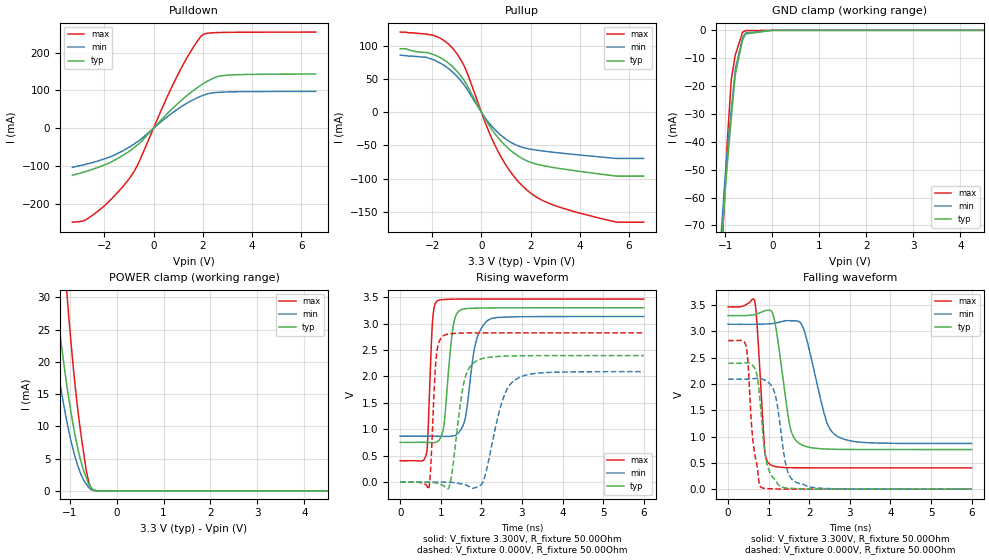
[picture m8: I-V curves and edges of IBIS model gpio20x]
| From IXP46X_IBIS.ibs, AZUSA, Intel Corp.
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[Model]   gpio20x
Model_type   I/O
Vinl = 800.000mV
Vinh = 2.000V
Vmeas = 1.500V
Cref = 0.000F
|   typ   min   max
C_comp   3.000pF   2.700pF   3.300pF
[Voltage Range]   3.300V   3.135V   3.465V
[Temperature Range]   25.0   110.0   -40.0
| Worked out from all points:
|   slope of the pulldown table from 0 to 0.495 V, typ, clamps not added: 14.5 ohm
|   slope of the pullup table from 0 to 0.495 V, typ, clamps not added: 16.7 ohm
|   POWER clamp passes 1 mA (typ) near -0.59 V on its own axis
|   falling waveform, V_fixture 3.300V, R_fixture 50.00Ohm: 20-80 % time 276ps typ, 421ps min, 141ps max; typ from 3.3 V to 0.753 V
|   rising waveform, V_fixture 3.300V, R_fixture 50.00Ohm: 20-80 % time 173ps typ, 247ps min, 92.3ps max; typ from 0.753 V to 3.3 V
|   rising waveform, V_fixture 0.000V, R_fixture 50.00Ohm: 20-80 % time 254ps typ, 400ps min, 105ps max; typ from 0 V to 2.4 V
|   falling waveform, V_fixture 0.000V, R_fixture 50.00Ohm: 20-80 % time 203ps typ, 243ps min, 179ps max; typ from 2.4 V to 0 V
[Pulldown]
|   Voltage   I(typ)   I(min)   I(max)
-3.3V     -124.6mA   -103.5mA   -248.9mA
-2.755V   -114.7mA   -95.53mA   -242.6mA
-2.29V    -104.7mA   -87.33mA   -221.2mA
-1.635V   -86.44mA   -72.55mA   -182.3mA
-925mV    -58.32mA   -47.76mA   -127.9mA
-605mV    -41.95mA   -33.66mA   -91.57mA
940mV     62.44mA    48.6mA     135.3mA
1.535V    95.49mA    72.67mA    205.6mA
1.99V     116.4mA    86.38mA    247mA
2.545V    135.5mA    94.53mA    253.1mA
2.875V    139.7mA    95.72mA    253.6mA
6.595V    143.5mA    97.58mA    254.5mA
[GND Clamp]
|   Voltage   I(typ)   I(min)   I(max)
-3.3V     -1.837A    -1.782A    -2.189A
-1.11V    -85mA      -78.05mA   -94.07mA
-1.015V   -60.26mA   -54.83mA   -58.33mA
-985mV    -53.42mA   -48.7mA    -48.27mA
-960mV    -48.28mA   -43.8mA    -39.96mA
-875mV    -31.55mA   -28.61mA   -17.72mA
-785mV    -15.46mA   -13.66mA   -8.602mA
-635mV    -3.516mA   -2.727mA   -731.7uA
-580mV    -1.636mA   -1.201mA   -155.8uA
-565mV    -1.289mA   -945.2uA   -102.2uA
0V        -56.84nA   -17.58nA   -565.5pA
6.595V    0A         0A         0A
[Pullup]
|   Voltage   I(typ)   I(min)   I(max)
-3.3V     95.67mA    85.92mA    120.8mA
-1.9V     86.2mA     78.19mA    115.1mA
-1.07V    64.88mA    56.95mA    91.89mA
-630mV    43.49mA    37.35mA    63.71mA
215mV     -13.96mA   -11.5mA    -21.37mA
695mV     -39.16mA   -31.53mA   -60.4mA
1.28V     -60.49mA   -47.08mA   -94.76mA
1.945V    -74.73mA   -55.41mA   -120.4mA
2.785V    -82.49mA   -59.82mA   -138mA
3.84V     -88.43mA   -63.94mA   -150.6mA
5.5V      -96.34mA   -69.74mA   -165.7mA
6.595V    -96.34mA   -69.74mA   -165.8mA
[POWER Clamp]
|   Voltage   I(typ)   I(min)   I(max)
-3.3V     221.1mA    178.3mA    361mA
-1.5V     44.33mA    31.93mA    79.94mA
-1.43V    39.23mA    27.99mA    71.16mA
-1.32V    31.69mA    22.21mA    58.04mA
-1.285V   29.42mA    20.49mA    54.06mA
-1.06V    16.5mA     10.87mA    30.94mA
-895mV    9.117mA    5.612mA    17.32mA
-780mV    5.203mA    2.981mA    10mA
-640mV    2mA        1.037mA    3.043mA
-540mV    479.4uA    207uA      465.4uA
-390mV    28.44uA    11.22uA    5.344uA
6.595V    0A         0A         0A
[Ramp]
R_load = 50.00Ohm
|   typ   min   max
dV/dt_r   1.437V/253.238ps   1.255V/399.378ps   1.695V/105.276ps
dV/dt_f   1.528V/275.536ps   1.360V/419.826ps   1.836V/140.921ps
[Falling Waveform]
V_fixture = 3.300V
V_fixture_min = 3.135V
V_fixture_max = 3.465V
R_fixture = 50.00Ohm
|   Time   V(typ)   V(min)   V(max)
0s        3.3V       3.135V     3.465V
650ps     3.32V      3.135V     3.588V
900ps     3.392V     3.139V     760.5mV
1.04ns    3.398V     3.144V     466mV
1.18ns    3.051V     3.159V     428.1mV
1.53ns    1.173V     3.202V     408.5mV
1.74ns    876.5mV    3.19V      406.7mV
2.43ns    762.2mV    1.276V     405mV
2.68ns    757.2mV    1.01V      404.9mV
6ns       753.2mV    868.8mV    404.9mV
[Rising Waveform]
V_fixture = 3.300V
V_fixture_min = 3.135V
V_fixture_max = 3.465V
R_fixture = 50.00Ohm
|   Time   V(typ)   V(min)   V(max)
0s        753.2mV    868.8mV    404.9mV
650ps     752.5mV    869.3mV    553.4mV
790ps     749.1mV    869.6mV    2.972V
910ps     764.3mV    869.1mV    3.428V
1.07ns    1.043V     866mV      3.455V
1.29ns    2.874V     871.9mV    3.463V
1.46ns    3.245V     957.3mV    3.464V
1.87ns    3.293V     2.668V     3.465V
2.2ns     3.298V     3.082V     3.465V
6ns       3.3V       3.135V     3.465V
[Rising Waveform]
V_fixture = 0.000V
V_fixture_min = 0.000V
V_fixture_max = 0.000V
R_fixture = 50.00Ohm
|   Time   V(typ)   V(min)   V(max)
0s        621.4nV    230.9nV    -1.797nV
700ps     157.6uV    -1.182uV   -131.4mV
890ps     -17.2mV    536.3uV    2.385V
1.07ns    -70.45mV   142.5uV    2.773V
1.21ns    -84.38mV   -2.132mV   2.806V
1.56ns    1.851V     -43.35mV   2.823V
1.83ns    2.27V      -109.2mV   2.824V
2.05ns    2.343V     25.1mV     2.825V
2.81ns    2.389V     1.926V     2.825V
6ns       2.395V     2.092V     2.825V
[Falling Waveform]
V_fixture = 0.000V
V_fixture_min = 0.000V
V_fixture_max = 0.000V
R_fixture = 50.00Ohm
|   Time   V(typ)   V(min)   V(max)
0s        2.395V     2.092V     2.825V
440ps     2.403V     2.091V     2.723V
610ps     2.349V     2.101V     924.8mV
720ps     2.123V     2.105V     405.4mV
820ps     1.366V     2.096V     31.8mV
1.03ns    315.2mV    2.002V     7.975mV
1.18ns    149.4mV    1.726V     4.125mV
1.44ns    22.72mV    405.6mV    1.245mV
1.69ns    10.03mV    126.2mV    282.1uV
6ns       621.4nV    230.9nV    -1.797nV
